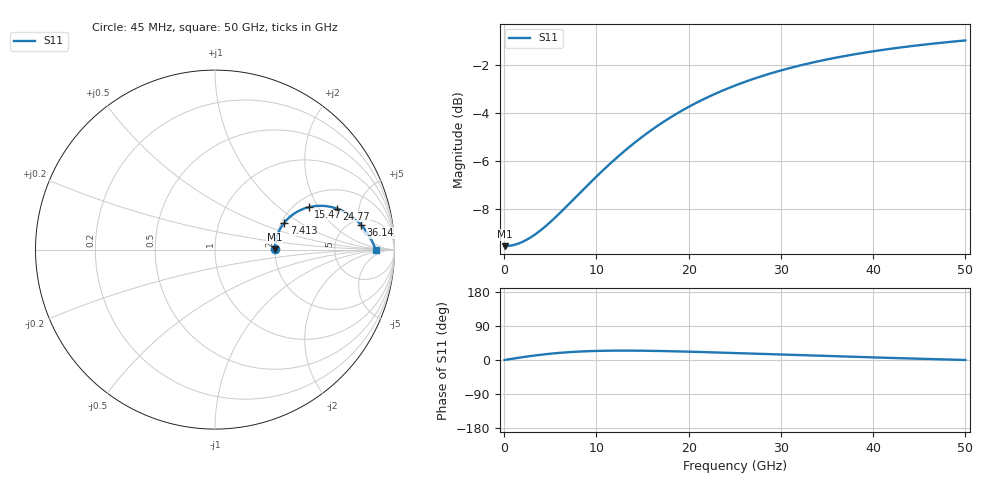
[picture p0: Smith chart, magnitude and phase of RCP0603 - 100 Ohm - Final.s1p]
!Vishay Electro-Films Inc.
!RCP Family
!Case Size 0603
!Assembly Style Surface Mount
!11/2/2015
!efi@vishay.com
# GHz S MA R 50
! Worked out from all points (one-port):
!   801 points, 45 MHz to 50 GHz, reference 50 ohm
!   lowest |S11| = -9.5 dB at 45 MHz (marker M1), VSWR 2.00, Z = 100 + j0.226 ohm
!   |S11| at or under -10 dB: nowhere
!   S11 on the Smith chart (normalised r, x): 45 MHz: 2.00, +0.00; 7.413 GHz: 2.08, +0.76; 15.47 GHz: 2.36, +1.66; 24.77 GHz: 3.15, +2.96; 36.14 GHz: 5.90, +5.12; 50 GHz: 18, +0
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0.045  0.3333 0.2
0.294775  0.3335 1.1
1.356319  0.3366 5.1
2.792525  0.3469 10.2
4.353619  0.365 14.9
6.289375  0.3951 19.4
7.413362  0.4152 21.3
8.724681  0.4402 22.9
9.973556  0.465 23.9
11.28487  0.4913 24.6
12.53375  0.5162 24.8
13.96996  0.5444 24.7
15.46861  0.5728 24.4
17.09214  0.6022 23.7
18.77812  0.6309 22.8
20.21433  0.6538 21.9
21.65054  0.6753 20.9
24.77273  0.7174 18.5
25.0225  0.7205 18.3
28.14469  0.7561 15.9
31.26687  0.7864 13.4
33.70218  0.8069 11.5
36.13749  0.8249 9.7
37.51125  0.8341 8.7
40.57099  0.8525 6.4
43.75563  0.8689 4.2
46.94026  0.883 2.0
50  0.8946 0.0
